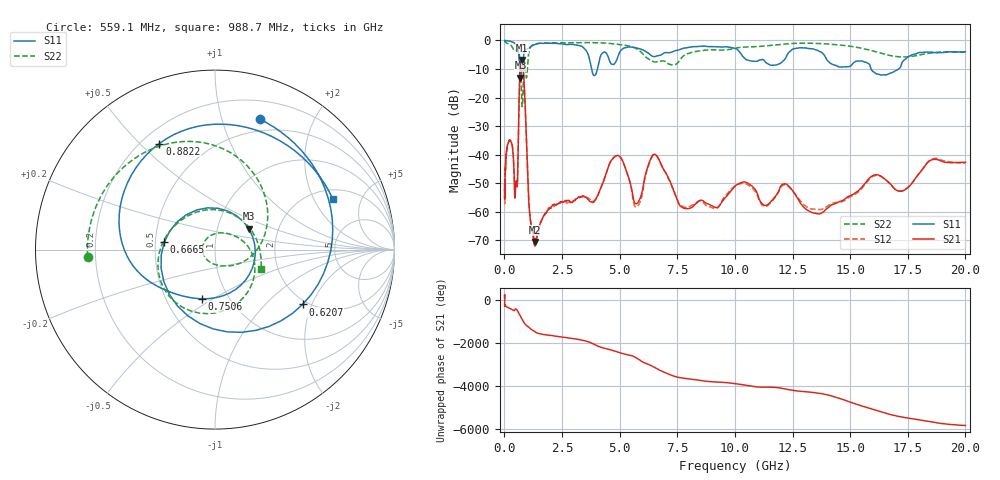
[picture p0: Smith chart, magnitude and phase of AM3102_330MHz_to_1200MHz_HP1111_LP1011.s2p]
! Date/Time: Tue, Sep 11, 2018 5:24 PM
! Network Analyzer: Agilent Technologies E8362B Rev: A.07.50.63
! Sweep from 0.010 to 20.000 GHz, 1601 Points, Sweep Type: LOG
! Power Supply: 4.949 V, 0.001 A
# Hz S DB R 50
!freq MagS11 AngS11 MagS21 AngS21 MagS12 AngS12 MagS22 AngS22
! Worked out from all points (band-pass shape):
!   1601 points, 10 MHz to 20 GHz, reference 50 ohm
!   highest |S21| = -6.81 dB at 747 MHz (marker M1); lowest = -70.5 dB at 1.334 GHz (marker M2)
!   |S21| within 3 dB of the highest: 685.6 MHz to 814.4 MHz (128.8 MHz wide, 17.2 % of centre)
!   lowest |S11| = -13.1 dB at 699 MHz (marker M3), VSWR 1.57, Z = 70.8 + j17.3 ohm
!   |S11| at or under -10 dB: 660.5 MHz to 765.2 MHz (104.7 MHz wide, 14.7 % of centre); 3.784 GHz to 4.037 GHz (253.4 MHz wide, 6.48 % of centre); 15.91 GHz to 17.1 GHz (1.194 GHz wide, 7.23 % of centre)
!   |S22| runs from -23.2 to -0.2 dB; largest |S21 - S12| = 0.0049
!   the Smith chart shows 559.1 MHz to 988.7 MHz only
!   S11 on the Smith chart (normalised r, x): 559.1 MHz: 0.38, +1.34; 620.7 MHz: 1.88, -1.72; 666.5 MHz: 0.56, +0.05; 750.6 MHz: 0.75, -0.45; 882.2 MHz: 0.27, +0.57; 988.7 MHz: 2.48, +2.86
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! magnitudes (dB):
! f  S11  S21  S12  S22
! 10 MHz  0.0  -52.5  -50.9  -0.2
! 35.55 MHz  -0.1  -46.4  -46.9  -0.5
! 126.4 MHz  -0.2  -37.0  -37.0  -1.0
! 336.3 MHz  -0.6  -36.7  -36.5  -2.3
! 447.2 MHz  -1.0  -54.1  -54.4  -3.8
! 559.1 MHz  -2.3  -50.7  -51.0  -3.0
! 620.7 MHz  -4.8  -27.6  -27.8  -3.6
! 666.5 MHz  -10.9  -13.0  -13.0  -6.2
! 699 MHz  -13.1  -8.5  -8.5  -9.8
! 747 MHz  -11.2  -6.8  -6.9  -19.1
! 750.6 MHz  -11.0  -6.8  -6.9  -20.1
! 882.2 MHz  -3.5  -19.1  -19.2  -8.7
! 988.7 MHz  -2.9  -42.2  -42.3  -11.1
! 1.334 GHz  -1.4  -70.5  -72.1  -1.2
! 1.59 GHz  -1.0  -63.3  -63.5  -1.0
! 3.865 GHz  -12.1  -56.6  -56.3  -0.8
! 4.855 GHz  -7.2  -40.4  -40.4  -1.3
! 5.652 GHz  -2.5  -56.8  -58.0  -2.6
! 6.518 GHz  -5.7  -39.8  -40.0  -7.5
! 7.845 GHz  -2.7  -58.9  -58.5  -5.0
! 13.55 GHz  -3.4  -60.7  -59.2  -1.1
! 20 GHz  -4.0  -42.6  -43.1  -4.1
